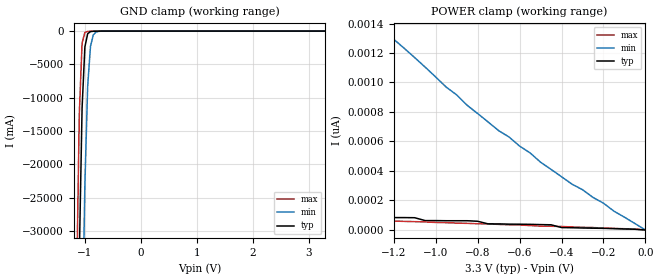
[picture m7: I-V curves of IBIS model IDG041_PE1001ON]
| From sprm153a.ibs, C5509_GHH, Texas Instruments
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| Pin_model   IDG041_PE1001ON
[Model]   IDG041_PE1001ON
 Model_type   Input
 Polarity   Non-Inverting
 Vinl  =  1.08
 Vinh  =  2.10
|Variable   typ   min   max
 C_comp   2.073pF   2.058pF   2.151pF
[Temperature Range]   25   125   -40
[Voltage Range]   3.3   3.0   3.6
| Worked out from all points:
|   GND clamp passes 1 mA (typ) near -0.59 V on its own axis
[GND Clamp]
|Voltage   I(typ)   I(min)   I(max)
-3.3V     -2.127kA   -2.167kA   -2.109kA
-1.15V    -66.48A    -117.1A    -39.31A
-1.1V     -33.84A    -80.11A    -12.46A
-1.05V    -11.54A    -47.82A    -1.806A
-1V       -2.382A    -22.98A    -205.2mA
-950mV    -392.2mA   -8.238A    -52.17mA
-900mV    -76.28mA   -2.294A    -31.66mA
-850mV    -25.66mA   -572.5mA   -22.84mA
-800mV    -14.09mA   -143.2mA   -15.74mA
-600mV    -1.097mA   -2.271mA   -800.6uA
3.3V      100.3uA    51.27uA    180.8uA
[POWER Clamp]
|Voltage   I(typ)   I(min)   I(max)
-3.3V     333.5pA    6.199nA    201.2pA
-3.25V    322.8pA    6.004nA    180.7pA
-3.05V    288.2pA    5.326nA    180.7pA
-3V       288.2pA    5.155nA    155.9pA
-2.7V     231.4pA    4.261nA    155pA
-2.5V     215.4pA    3.745nA    123.9pA
-1.8V     137.2pA    2.246nA    108.8pA
-1.75V    137.2pA    2.156nA    81.27pA
-1.25V    83.93pA    1.37nA     61.73pA
-700mV    41.3pA     673.7pA    37.75pA
-350mV    15.1pA     310.4pA    20.43pA
0V        0A         0A         0A
